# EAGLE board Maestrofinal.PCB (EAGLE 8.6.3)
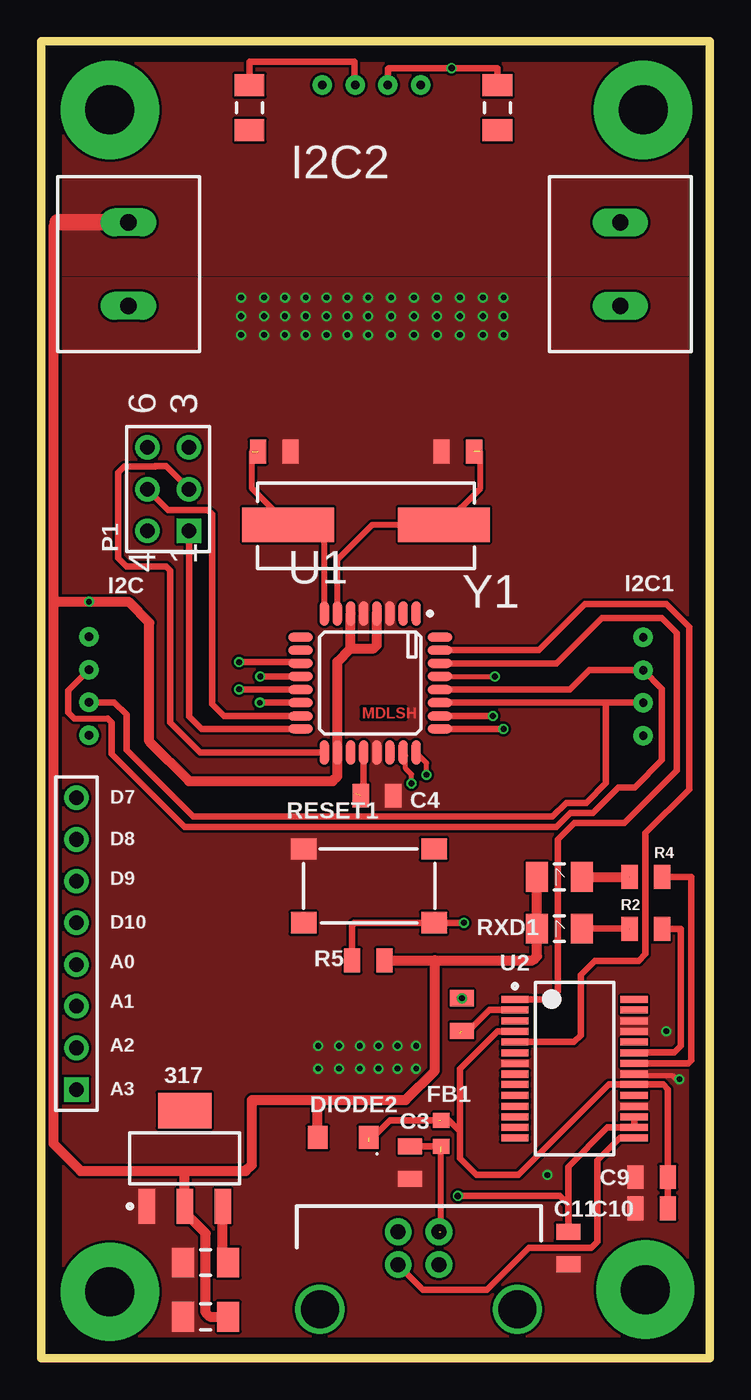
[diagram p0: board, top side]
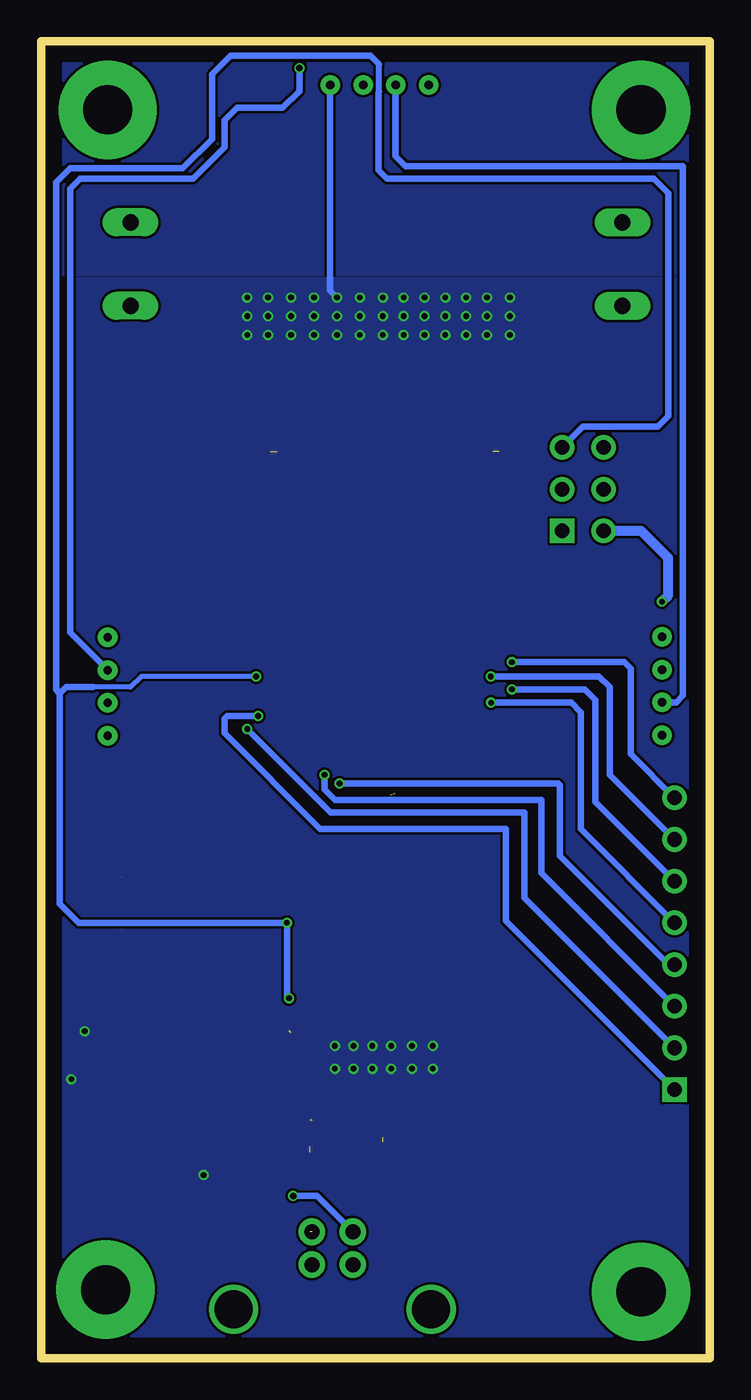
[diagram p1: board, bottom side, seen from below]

Size 40.77 x 80.26 mm. Coordinates in mm from the lower left corner, seen from the top.
Outline: 0,0 0,80.26 40.77,80.26 40.77,0 0,0
Copper layers (1*16): Top 0.035mm / dielectric 1.5mm / Bottom 0.035mm
Design rules "Maestrofinal": minimum track width 6mil, minimum drill 0.35mm, track to track 6mil, track to pad 6mil, pad to pad 6mil, via to via 6mil, smd to smd 6mil, copper to edge 40mil, drill to drill 6mil, minimum pad ring 0mil, minimum via ring 0mil, stop-mask expansion 4mil, vias tented up to drill 0mil, thermal gap 10mil

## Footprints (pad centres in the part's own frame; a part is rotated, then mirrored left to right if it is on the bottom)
SOT230P700X180-4N_1PRIMARY = smd 2.159 x 0.991: 1 -2.921,2.311; 2 -2.921,0; 3 -2.921,-2.311 | smd 2.159 x 3.251: 4 2.921,0
CAPC0805-I_1PRIMARY = smd 0.991 x 1.448: 1 -0.991,0; 2 0.991,0
CAPC0805_1PRIMARY = smd 0.991 x 1.448: 1 -0.991,0; 2 0.991,0
CAPC1206_1PRIMARY = smd 1.346 x 1.803: 1 -1.372,0; 2 1.372,0
SODFL360X143-2N_1PRIMARY = smd 1.194 x 1.397: 1 -1.549,0; 2 1.549,0
IND0603_1PRIMARY = smd 0.914 x 0.991: 1 -0.787,0; 2 0.787,0
GROVE90_1PRIMARY = drill 0.508 pad 1.194: 1 -2.997,0; 2 -0.991,0; 3 0.991,0; 4 2.997,0
2PIN_1PRIMARY = drill 0.991 pad 1.702 long: 1 0,0; 2 5.08,0
HDR2X3_CEN_1PRIMARY = drill 0.889 pad 1.499 square: 1 0,0 | drill 0.889 pad 1.499: 2 2.54,0; 3 5.08,0; 4 0,2.54; 5 2.54,2.54; 6 5.08,2.54
HDR1X8_1PRIMARY = drill 0.889 pad 1.499 square: 1 0,0 | drill 0.889 pad 1.499: 2 2.54,0; 3 5.08,0; 4 7.62,0; 5 10.16,0; 6 12.7,0; 7 15.24,0; 8 17.78,0
RESC1206_1PRIMARY = smd 1.346 x 1.803: 1 -1.372,0; 2 1.372,0
RESC0805_1PRIMARY = smd 0.991 x 1.448: 1 -0.991,0; 2 0.991,0
RESC0805-I_1PRIMARY = smd 0.991 x 1.448: 1 -0.991,0; 2 0.991,0
BUTTON_1PRIMARY = smd 1.549 x 1.295: 1 0,0; 2 7.95,0; 3 0,-4.496; 4 7.95,-4.496
LED1206_1PRIMARY = smd 1.346 x 1.803: 1 -1.372,0; 2 1.372,0
TQFP-32_1PRIMARY = smd 1.499 x 0.559: 1 -4.242,2.794; 2 -4.242,2.007; 3 -4.242,1.194; 4 -4.242,0.406; 5 -4.242,-0.406; 6 -4.242,-1.194; 7 -4.242,-2.007; 8 -4.242,-2.794; 17 4.242,-2.794; 18 4.242,-2.007; 19 4.242,-1.194; 20 4.242,-0.406; 21 4.242,0.406; 22 4.242,1.194; 23 4.242,2.007; 24 4.242,2.794 | smd 0.559 x 1.499: 9 -2.794,-4.242; 10 -2.007,-4.242; 11 -1.194,-4.242; 12 -0.406,-4.242; 13 0.406,-4.242; 14 1.194,-4.242; 15 2.007,-4.242; 16 2.794,-4.242; 25 2.794,4.242; 26 2.007,4.242; 27 1.194,4.242; 28 0.406,4.242; 29 -0.406,4.242; 30 -1.194,4.242; 31 -2.007,4.242; 32 -2.794,4.242
TSSOP-28_1PRIMARY = smd 1.651 x 0.432: 1 -3.632,4.216; 2 -3.632,3.581; 3 -3.632,2.921; 4 -3.632,2.286; 5 -3.632,1.626; 6 -3.632,0.965; 7 -3.632,0.33; 8 -3.632,-0.33; 9 -3.632,-0.965; 10 -3.632,-1.626; 11 -3.632,-2.286; 12 -3.632,-2.921; 13 -3.632,-3.581; 14 -3.632,-4.216; 15 3.632,-4.216; 16 3.632,-3.581; 17 3.632,-2.921; 18 3.632,-2.286; 19 3.632,-1.626; 20 3.632,-0.965; 21 3.632,-0.33; 22 3.632,0.33; 23 3.632,0.965; 24 3.632,1.626; 25 3.632,2.286; 26 3.632,2.921; 27 3.632,3.581; 28 3.632,4.216
USB_B_1PRIMARY = drill 0.914 pad 1.626: 1 -1.245,0; 2 -1.245,2.007; 3 1.245,0; 6 1.245,2.007 | drill 2.311 pad 2.997: 4 6.02,-2.718; 5 -6.02,-2.718
HC49/US_1PRIMARY = smd 5.588 x 2.108: 1 -4.75,0; 2 4.75,0

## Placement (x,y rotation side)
317  [SOT230P700X180-4N_1PRIMARY]  8.76,12.19 90 top
C1  [CAPC0805-I_1PRIMARY]  14.22,55.25 180 top
C2  [CAPC0805-I_1PRIMARY]  25.4,55.25 0 top
C3  10nF  [CAPC0805_1PRIMARY]  22.48,11.94 90 top
C4  100nF  [CAPC0805_1PRIMARY]  20.47,34.29 0 top
C5  [CAPC1206_1PRIMARY]  10.03,5.84 0 top
C6  [CAPC1206_1PRIMARY]  10.03,2.54 0 top
C8  100nF  [CAPC0805_1PRIMARY]  25.65,20.96 270 top
C9  100nF  [CAPC0805_1PRIMARY]  37.21,11.05 0 top
C10  4.7uF  [CAPC0805_1PRIMARY]  37.21,9.14 0 top
C11  100nF  [CAPC0805_1PRIMARY]  32.13,6.73 90 top
DIODE2  SS1P3L  [SODFL360X143-2N_1PRIMARY]  18.41,13.46 180 top
FB1  FerriteBead  [IND0603_1PRIMARY]  24.38,13.72 90 top
I2C  Grove_I2C  [GROVE90_1PRIMARY]  2.92,40.97 90 top
I2C1  Grove_I2C2  [GROVE90_1PRIMARY]  36.7,40.94 90 top
I2C2  Grove_I2C2  [GROVE90_1PRIMARY]  20.14,77.6 0 top
INPUT  [2PIN_1PRIMARY]  5.33,69.22 270 top
OUTPUT  [2PIN_1PRIMARY]  35.31,64.14 90 top
P1  Header_3X2A  [HDR2X3_CEN_1PRIMARY]  9.02,50.42 90 top
P5  D/A  [HDR1X8_1PRIMARY]  2.16,16.38 90 top
R1  [RESC1206_1PRIMARY]  27.81,76.2 270 top
R2  270  [RESC0805_1PRIMARY]  36.86,26.16 0 top
R3  [RESC1206_1PRIMARY]  12.7,76.2 270 top
R4  270  [RESC0805_1PRIMARY]  36.86,29.34 0 top
R5  1k  [RESC0805-I_1PRIMARY]  19.94,24.26 180 top
RESET1  [BUTTON_1PRIMARY]  16,31.04 0 top
RXD1  [LED1206_1PRIMARY]  31.6,26.19 0 top
TXD1  [LED1206_1PRIMARY]  31.6,29.34 0 top
U1  ATmega328P-AU  [TQFP-32_1PRIMARY]  20.07,41.15 270 top
U2  FT232RL-Reel  [TSSOP-28_1PRIMARY]  32.51,17.65 0 top
VBUS1  USB-B  [USB_B_1PRIMARY]  23.01,5.71 0 top
Y1  XTAL  [HC49/US_1PRIMARY]  19.81,50.8 0 top

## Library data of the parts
317 C1-C6 C8-C11 DIODE2 FB1 I2C I2C1 I2C2 INPUT OUTPUT P1 P5 R1-R5 RESET1 RXD1 TXD1 U1 U2 VBUS1 Y1 = Maestrofinal

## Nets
3V3: C11.2 U2.16 U2.17 VBUS1.2
5V: DIODE2.2 R5.1
A0: P5.4 U1.23
A1: P5.3 U1.24
A2: P5.2 U1.25
A3: P5.1 U1.26
D7: P5.8 U1.11
D8: P5.7 U1.12
D9: P5.6 U1.13
D10: P5.5 U1.14
GND: 317.1 C1.1 C2.1 C3.1 C4.2 C5.1 C6.1 C9.1 C10.1 C11.1 RESET1.1 U1.3 U1.5 U1.21 U2.7 U2.18 U2.21 U2.25 U2.26
MISO: P1.1 U1.16
MOSI: P1.5 U1.15
NETC1_2: C1.2 U1.8 Y1.1
NETC2_2: C2.2 U1.7 Y1.2
NETC3_2: C3.2 FB1.1 VBUS1.6
NETC4_1: C4.1 U1.20
NETC8_2: C8.2 U2.2
NETR2_1: R2.1
NETR2_2: R2.2 U2.23
NETR4_1: R4.1
NETR4_2: R4.2 U2.22
NETU2_15: U2.15 VBUS1.1
RESET: C8.1 P1.3 R5.2 RESET1.4 U1.29
RXD: U1.31 U2.5
SCK: P1.2 U1.17
SCL: R1.1 U1.28
SDA: R3.1 U1.27
TXD: U1.30 U2.1
VCC: 317.3 C5.2
VUSB: C9.2 C10.2 DIODE2.1 FB1.2 U2.4 U2.20

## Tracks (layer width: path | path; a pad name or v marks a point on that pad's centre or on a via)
3V3  (via drill 0.4 pad 0.61)
  Top 0.406: U2.17 U2.16 34.52,14.07 32.13,11.68 32.13,9.4 | v25.4,9.91 31.62,9.91 32.13,9.4 | C11.2 32.13,9.4
  Bottom 0.406: v25.4,9.91 23.95,9.91 VBUS1.2
5V  (via drill 0.35 pad 0.61)
  Top 0.61: 1.02,69.22 0.76,68.96 0.76,46.1 | R5.1 24,24.26 | 24,24.26 29.97,24.26 30.23,24.51 30.23,29.34 | 24,24.26 24,17.53 22.23,15.75 16.89,15.75 | 16.87,13.21 DIODE2.2 16.87,15.72 16.89,15.75 | 0.76,46.1 0.76,13.08 2.41,11.43 8.76,11.43 | 8.76,11.43 12.47,11.43 12.85,11.79 12.85,15.75 16.89,15.75 | 0.76,46.1 v2.92,46.1 5.33,46.1 6.6,44.83 6.6,37.59 9.02,35.18 17.78,35.18 18.06,35.46 18.06,42.44 18.87,43.26 | 8.76,11.43 8.76,8.89 10.03,7.62 10.03,2.79 10.29,2.54 11.41,2.54 | 20.47,45.39 20.47,43.46 20.27,43.26 18.87,43.26 | 18.87,43.26 18.87,45.39
  Top 1: 1.02,69.22 5.33,69.22
  Bottom 0.61: v2.92,46.1 2.54,46.48 2.54,48.77 4.19,50.42 6.48,50.42
  pour Top (no thermals): 0,66.04 0,80.26 40.77,80.26 40.77,66.04
  pour Bottom (no thermals): 0,80.26 0,66.04 40.77,66.04 40.77,80.26
A0  (via drill 0.35 pad 0.61)
  Top 0.305: v22.58,35.03 22.58,35.58 22.23,35.94 22.23,36.73 U1.23
  Bottom 0.305: 9.14,34.92 9.25,35.03
  Bottom 0.406: 9.25,35.03 v22.58,35.03 | 9.14,34.92 9.14,30.61 2.54,24 P5.4
A1  (via drill 0.35 pad 0.61)
  Top 0.305: v23.5,35.56 23.5,36.27 U1.24
  Bottom 0.406: v23.5,35.56 23.5,34.67 22.86,34.04 10.29,34.04 10.29,29.59 P5.3
A2  (via drill 0.35 pad 0.61)
  Top 0.406: U1.25 v28.19,38.35
  Bottom 0.406: P5.2 11.3,28.07 11.3,33.27 23.11,33.27 v28.19,38.35
A3  (via drill 0.35 pad 0.61)
  Top 0.406: U1.26 v27.53,39.14
  Bottom 0.406: v27.53,39.14 29.44,39.14 29.59,38.99 29.59,38.1 23.75,32.26 12.45,32.26 12.45,26.67 P5.1
D7  (via drill 0.35 pad 0.61)
  Top 0.406: v12.07,42.42 15.75,42.42 U1.11
  Bottom 0.406: v12.07,42.42 5.21,42.42 4.83,42.04 4.83,36.83 P5.8
D8  (via drill 0.35 pad 0.61)
  Top 0.406: v13.36,41.55 U1.12
  Bottom 0.406: P5.7 6.1,35.56 6.1,40.89 6.76,41.55 v13.36,41.55
D9  (via drill 0.35 pad 0.61)
  Top 0.406: v12.07,40.77 15.8,40.77 U1.13
  Bottom 0.406: v12.07,40.77 7.62,40.77 6.98,40.13 6.98,33.91 P5.6
D10  (via drill 0.35 pad 0.61)
  Top 0.406: v13.34,39.95 U1.14
  Bottom 0.406: v13.34,39.95 8.46,39.95 7.87,39.37 7.87,32.26 P5.5
GND  (via drill 0.35 pad 0.61)
  Top 0.305: v38.91,17.02 38.71,17.02 38.48,17.25 36.22,17.25 U2.21
  Bottom 0.406: v22.73,64.64 23.14,65.05 23.14,77.6
  other vias: 38.1,19.94 30.86,11.18 20.57,17.65 20.57,19.05 21.72,17.65 21.72,19.05 19.43,17.65 19.43,19.05 22.86,17.65 22.86,19.05 18.16,17.65 16.89,17.65 16.89,19.05 18.16,19.05 28.19,62.36 28.19,63.5 28.19,64.64 26.92,62.36 26.92,63.5 26.92,64.64 25.53,62.36 25.53,63.5 25.53,64.64 24.13,62.36 24.13,63.5 24.13,64.64 22.73,63.5 22.73,62.36 21.34,62.36 21.34,63.5 21.34,64.64 19.94,62.36 19.94,63.5 19.94,64.64 18.67,62.36 18.67,63.5 18.67,64.64 17.4,62.36 17.4,63.5 17.4,64.64 16.13,62.36 16.13,63.5 16.13,64.64 14.86,62.36 14.86,63.5 14.86,64.64 13.59,62.36 13.59,63.5 13.59,64.64 12.19,62.36 12.19,63.5 12.19,64.64
  pour Top (no thermals): 0.12,0.12 40.64,0.12 40.64,65.78 0.12,65.78
  pour Bottom (no thermals): 0.13,65.79 40.64,65.79 40.64,0.13 0.13,0.13
MISO
  Top 0.406: P1.1 9.02,39.12 9.78,38.35 U1.16
MOSI
  Top 0.406: U1.15 11.15,39.14 10.41,39.88 10.41,51.44 10.16,51.69 7.75,51.69 P1.5
NETC1_2  (1 unrouted)
  Top 0.356: 12.85,55.25 12.85,53.01 Y1.1 17.15,50.8 17.27,50.67 U1.8
NETC2_2  (1 unrouted)
  Top 0.356: 26.77,55.25 26.77,53.01 Y1.2 20.19,50.8 18.06,48.67 U1.7
NETC3_2  (2 unrouted)
  Top 0.356: 24.38,7.72 24.38,12.57
  Top 0.406: C3.2 FB1.1
NETC4_1  (1 unrouted)
  Top 0.406: 19.2,34.42 19.66,34.9 U1.20
NETC8_2  (1 unrouted)
  Top 0.406: 25.65,19.71 25.53,19.84 25.93,19.84 27.33,21.23 U2.2
NETR2_1  (1 unrouted)
  Top 0.406: 35.84,26.16 35.81,26.19 32.97,26.19
NETR2_2
  Top 0.406: U2.23 36.14,18.64 38.58,18.64 38.99,19.05 38.99,26.16 R2.2
NETR4_1  (1 unrouted)
  Top 0.61: 32.97,29.34 35.84,29.34
NETR4_2
  Top 0.406: U2.22 39.45,17.98 39.62,18.16 39.62,29.34 R4.2
NETU2_15
  Top 0.406: VBUS1.1 23.29,4.19 27.18,4.19 29.72,6.73 33.53,6.73 33.91,7.11 33.91,12.07 35.28,13.44 U2.15
RESET  (via drill 0.35 pad 0.61)
  Top 0.305: U1.29 v27.66,41.55
  Top 0.406: v25.78,26.54 RESET1.4 19.08,26.54 18.95,26.39 R5.2
  Bottom 0.305: 37.59,40.89 35.31,40.89 34.65,41.55 v27.66,41.55
  Bottom 0.356: 20.7,79.38 20.17,78.84 20.17,77.19 20.19,77.17 20.19,76.96
  Bottom 0.406: C8.1 25.76,21.95 25.78,21.97 v25.78,26.54 38.48,26.54 39.62,27.69 39.62,40.51 | 39.62,40.51 39.85,40.74 39.85,71.65 38.99,72.52 32.13,72.52 30.35,74.3 30.35,78.23 29.21,79.38 20.7,79.38 | 39.62,40.51 39.24,40.89 37.59,40.89 | 20.19,76.96 20.19,72.39 19.69,71.88 3.43,71.88 2.54,70.99 2.54,57.4 3.18,56.77 7.75,56.77 P1.3
  other vias: 25.65,21.95
RXD
  Top 0.406: U1.31 30.33,43.16 33.15,45.97 38.1,45.97 39.5,44.58 39.5,34.67 36.83,32 36.83,24.64 36.42,24.23 33.76,24.23 32.89,23.37 32.89,19.68 32.49,19.28 U2.5
S$1  (via drill 3 pad 5.99)
  other vias: 4.19,76.07
S$2  (via drill 3 pad 5.99)
  other vias: 36.7,76.07
S$3  (via drill 3 pad 5.99)
  other vias: 36.83,4.19
S$4  (via drill 3 pad 5.99)
  other vias: 4.19,4.06
SCK
  Top 0.406: U1.17 9.7,36.91 7.87,38.73 7.87,48.01 7.62,48.26 5.21,48.26 4.7,48.77 4.7,53.98 5.06,54.33 6.96,54.33 6.96,54.36 7.62,54.36 P1.2
SCL  (via drill 0.4 pad 0.61)  (1 unrouted)
  Top 0.356: 2.03,38.99 4.06,38.99
  Top 0.406: U1.28 32.23,40.74 33.43,41.94 36.7,41.94 37.85,40.79 37.85,36.45 36.2,34.8 35.18,34.8 33.63,33.25 32.26,33.25 31.39,32.39 8.76,32.39 4.32,36.83 4.32,38.73 4.06,38.99 | 2.03,38.99 1.65,39.37 1.65,40.69 2.92,41.96 | 21.13,77.6 21.13,78.56 21.21,78.61 v25.02,78.61 27.81,78.61 R1.1
  Bottom 0.406: v25.02,78.61 25.02,77.22 26.04,76.2 28.83,76.2 29.59,75.44 29.59,73.79 31.5,71.88 38.38,71.88 38.99,71.27 38.99,44.22 36.7,41.94
SDA  (2 unrouted)
  Top 0.254: 19.1,77.65 19.15,77.6 | U1.27 24.33,39.95
  Top 0.406: 19.1,77.65 19.1,78.99 12.7,78.99 R3.1 | 2.92,39.98 4.47,39.98 5.21,39.24 5.21,37.08 9.27,33.02 31.17,33.02 32,33.86 33.22,33.86 34.42,35.05 34.42,39.95 | 24.33,39.95 34.42,39.95 | 34.42,39.95 36.7,39.95
  Bottom 0.406: 19.15,77.6 19.15,73.25 18.54,72.64 1.65,72.64 1.65,40.39 2.06,39.98 2.92,39.98
TXD
  Top 0.406: U2.1 31.01,21.87 31.5,22.35 31.5,31.62 32.51,32.64 35.56,32.64 38.73,35.81 38.73,44.2 37.82,45.11 34.19,45.11 31.42,42.34 U1.30
VCC
  Top 0.61: C5.2 11.07,6.2 317.3
VUSB  (2 unrouted)
  Top 0.406: 19.96,13.21 21.26,14.5 24.26,14.5 | U2.4 27.81,19.94 25.53,17.65 25.53,13.84 | 25.53,13.84 25.53,12.19 26.54,11.18 29.08,11.18 34.59,16.69 U2.20 37.92,16.69 38.2,16.41 C9.2 C10.2 | 25.53,13.84 24.87,14.5 FB1.2

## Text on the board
Top: MDLSH
tPlace: D7 | D8 | D9 | D10 | A0 | A1 | A2 | A3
